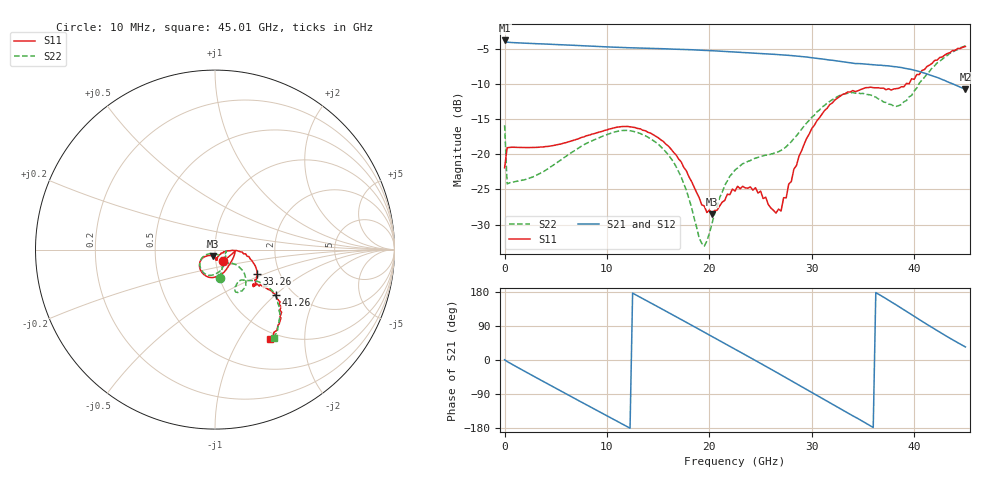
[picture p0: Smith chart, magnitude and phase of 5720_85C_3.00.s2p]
! Device:  ADRF5720
! Description: 0.5dB LSB GaAs MMIC 6-bit Digital Attenuator
! Frequency:  0.000009 -  40 GHz
! Ports:
!	RF1	= Port 1
!	RF2	= Port 2
! Vdd:  3.3 Volt
! Vss:  -3.3 Volt
! Control:  0/3.3 Volt
! State:  3.00 dB attenuation
! Data:  The device was measured using G-S-G Probes on a matrix board.
!  Data was collected using an calibrated 4 port network analyzer.
!  The reference plane for this measurement is at the launchers.
! Note:  Analog Devices supplies this data as a sample of measured data
!  for this product.  Your particular data for this product may vary.
!  Data was taken at 85 degrees C.
!  Analog Devices reserves the right to change this data at anytime.
# GHZ S DB R 45.0
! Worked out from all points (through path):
!   181 points, 10 MHz to 45.01 GHz, reference 45 ohm
!   highest |S21| = -3.80 dB at 10 MHz (marker M1); lowest = -10.8 dB at 45.01 GHz (marker M2)
!   group delay of S21, straight-line fit = 42 ps
!   lowest |S11| = -28.5 dB at 20.26 GHz (marker M3), VSWR 1.08, Z = 43.7 - j3.09 ohm
!   |S11| at or under -10 dB: start of sweep to 39.21 GHz
!   |S22| runs from -33.1 to -4.5 dB; largest |S21 - S12| = 0.0034
!   S11 on the Smith chart (normalised r, x): 10 MHz: 1.09, -0.14; 33.26 GHz: 1.53, -0.44; 41.26 GHz: 1.64, -1.00; 45.01 GHz: 0.90, -1.36
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0.01  -21.92 -55.4  -3.80 0.6  -3.78 0.6  -15.87 -79.9
0.26  -19.07 -5.4  -4.05 -4.0  -4.04 -4.0  -24.22 -7.2
2.01  -19.04 -20.1  -4.19 -30.4  -4.17 -30.4  -23.61 -21.2
4.26  -18.88 -41.6  -4.33 -63.6  -4.31 -63.5  -22.05 -45.8
7.76  -17.52 -66.1  -4.56 -114.7  -4.54 -114.7  -18.65 -72.3
11.51  -16.05 -98.2  -4.80 -169.1  -4.79 -169.0  -16.61 -104.3
15.26  -17.94 -132.8  -4.97 136.3  -4.95 136.4  -18.91 -137.8
17.26  -21.09 -145.2  -5.07 106.8  -5.05 107.0  -23.24 -150.2
19.26  -27.19 -132.2  -5.19 77.1  -5.17 77.3  -32.67 -110.4
20.26  -28.50 -110.2  -5.26 62.1  -5.24 62.3  -29.87 -60.6
21.51  -26.56 -85.0  -5.36 43.5  -5.35 43.7  -24.41 -51.0
22.76  -24.55 -80.7  -5.47 24.8  -5.45 25.1  -21.96 -53.6
24.76  -25.52 -81.5  -5.64 -5.2  -5.62 -4.9  -20.42 -57.2
27.01  -28.07 -28.9  -5.84 -39.4  -5.82 -39.1  -19.44 -44.5
28.26  -22.11 -4.5  -5.99 -58.7  -5.97 -58.4  -17.75 -37.8
30.26  -15.87 -8.4  -6.30 -89.7  -6.28 -89.4  -14.44 -37.0
33.26  -11.39 -30.0  -6.87 -135.9  -6.85 -135.5  -11.39 -52.2
35.51  -10.51 -41.6  -7.19 -170.2  -7.17 -169.9  -11.50 -63.3
37.76  -10.86 -41.9  -7.47 153.5  -7.45 153.9  -12.92 -56.9
39.26  -9.90 -39.5  -7.81 128.0  -7.79 128.4  -12.35 -44.8
41.26  -7.50 -36.5  -8.56 94.0  -8.54 94.4  -8.60 -35.3
45.01  -4.66 -58.6  -10.76 34.5  -10.73 34.8  -4.55 -56.1
